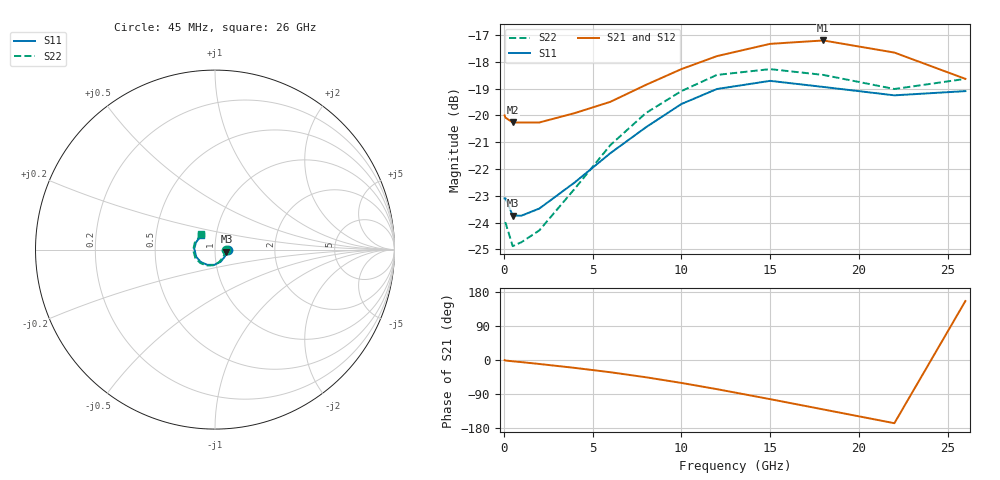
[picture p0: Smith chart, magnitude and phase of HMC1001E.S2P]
! HMMC-1001
! Typical s-parameters at 20dB attenuator setting, TA = 25 C
# ghz s ma r 50
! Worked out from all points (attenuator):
!   14 points, 45 MHz to 26 GHz, reference 50 ohm
!   highest |S21| = -17.20 dB at 18 GHz (marker M1); lowest = -20.3 dB at 500 MHz (marker M2)
!   lowest |S11| = -23.7 dB at 500 MHz (marker M3), VSWR 1.14, Z = 56.8 - j1.3 ohm
!   |S11| at or under -10 dB: start of sweep to end of sweep
!   |S22| runs from -24.9 to -18.3 dB; largest |S21 - S12| = 0.0027
0.045  0.07 -1.5  0.1 -0.4  0.1 -0.5  0.063 -2.0
0.1  0.07 -4.0  0.099 -1.4  0.099 -1.6  0.063 -5.1
0.5  0.065 -10.1  0.097 -3.4  0.097 -3.1  0.057 -11.4
1  0.065 -17.7  0.097 -5.6  0.096 -5.4  0.058 -20.6
2  0.067 -33.8  0.097 -10.5  0.097 -10.6  0.061 -38.6
4  0.075 -64.6  0.101 -20.8  0.1 -20.8  0.073 -70.7
6  0.085 -92.2  0.106 -32.3  0.107 -32.3  0.088 -96.3
8  0.095 -116.6  0.114 -45.5  0.114 -45.7  0.101 -118.6
10  0.105 -138.7  0.122 -60.5  0.122 -60.7  0.111 -138.1
12  0.112 -158.3  0.129 -76.9  0.129 -76.8  0.119 -156.2
15  0.116 176.9  0.136 -103.3  0.136 -103.1  0.122 -178.9
18  0.113 158.7  0.138 -130.5  0.136 -130.5  0.119 161.6
22  0.109 145.8  0.131 -166.8  0.132 -167.9  0.112 145.1
26  0.111 133.6  0.117 155.6  0.117 155.2  0.117 131.6
